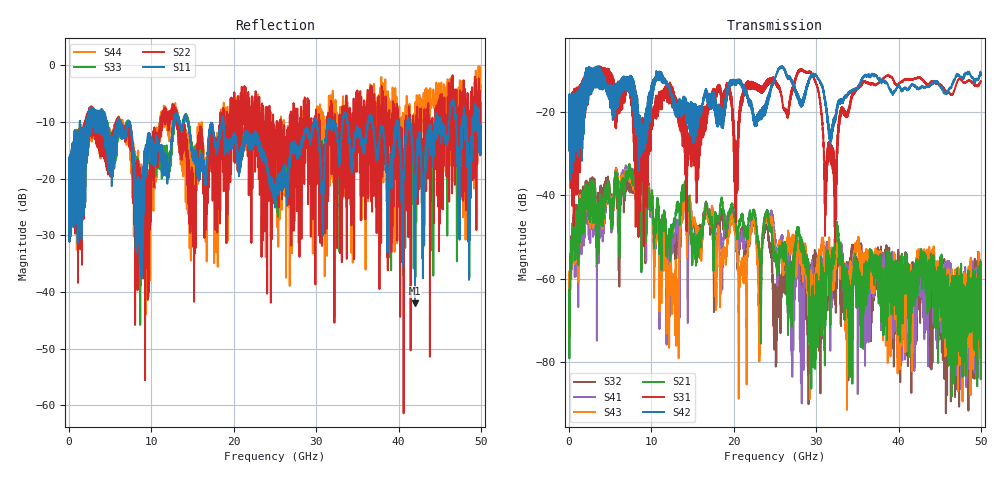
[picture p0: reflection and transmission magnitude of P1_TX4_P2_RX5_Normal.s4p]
!Keysight Technologies,N5225B,MY57041031,A.13.20.10
!Date: Friday, May 31, 2019 11:35:19
!Correction: S11(Full 4 Port(1,2,3,4))
!S12(Full 4 Port(1,2,3,4))
!S13(Full 4 Port(1,2,3,4))
!S14(Full 4 Port(1,2,3,4))
!S21(Full 4 Port(1,2,3,4))
!S22(Full 4 Port(1,2,3,4))
!S23(Full 4 Port(1,2,3,4))
!S24(Full 4 Port(1,2,3,4))
!S31(Full 4 Port(1,2,3,4))
!S32(Full 4 Port(1,2,3,4))
!S33(Full 4 Port(1,2,3,4))
!S34(Full 4 Port(1,2,3,4))
!S41(Full 4 Port(1,2,3,4))
!S42(Full 4 Port(1,2,3,4))
!S43(Full 4 Port(1,2,3,4))
!S44(Full 4 Port(1,2,3,4))
!S4P File: Measurements: <S11,S12,S13,S14>,
!<S21,S22,S23,S24>,
!<S31,S32,S33,S34>,
!<S41,S42,S43,S44>:
# Hz S  dB  R 50.0
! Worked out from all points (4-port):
!   5000 points, 10 MHz to 50 GHz, reference 50 ohm
!   strongest paths, dB at 10 MHz, 12.51 GHz, 25.01 GHz, 37.51 GHz, 50 GHz:
!     S42: -19.5, -16.9, -11.8, -11.9, -11.1
!     S31: -19.6, -17.6, -12.9, -13.1, -12.6
!     S21: -67.5, -48.5, -55.1, -58.6, -61.4
!     S43: -58.3, -60.5, -54.2, -54.2, -61.3
!     S41: -63.3, -52.4, -50.4, -58.5, -59.8
!     S32: -67.7, -51.0, -61.5, -53.8, -68.4
!   lowest |S11| = -42.0 dB at 42 GHz (marker M1), VSWR 1.02, Z = 49.3 + j0.299 ohm
!   |S11| at or under -10 dB: 7.336 GHz to 12.7 GHz (5.362 GHz wide, 53.5 % of centre); 14.41 GHz to 18.57 GHz (4.157 GHz wide, 25.2 % of centre); 18.74 GHz to 29.76 GHz (11.02 GHz wide, 45.4 % of centre)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
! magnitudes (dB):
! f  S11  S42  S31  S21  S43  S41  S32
! 10 MHz  -19.6  -19.5  -19.6  -67.5  -58.3  -63.3  -67.7
! 7.37 GHz  -10.1  -13.9  -14.5  -32.7  -35.5  -33.2  -37.8
! 13.07 GHz  -9.5  -18.3  -17.8  -42.2  -64.6  -46.0  -51.0
! 13.94 GHz  -9.3  -18.8  -28.3  -38.1  -40.5  -40.0  -40.9
! 29.46 GHz  -11.9  -11.0  -10.8  -66.2  -62.1  -59.8  -56.2
! 42 GHz  -42.0  -13.5  -11.9  -59.6  -63.5  -59.3  -81.1
! 50 GHz  -12.1  -11.1  -12.6  -61.4  -61.3  -59.8  -68.4
